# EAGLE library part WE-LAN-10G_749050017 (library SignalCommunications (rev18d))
WE-LAN 10G Transformer 10Gbit Base-T - Compliant with standards: IEEE 802.3an and upcoming IEEE 802.3bt - SMD -- Ethernet -- Ethernet speed up to 10Gbit/s --Power over Ethernet PoE and PoE+ --10Gbit with ETR and PoE up to 150 W (for industrial applications) Details see: http://katalog.we-online.de/en/pbs/WE-LAN-10G 2015 (C) Würth Elektronik
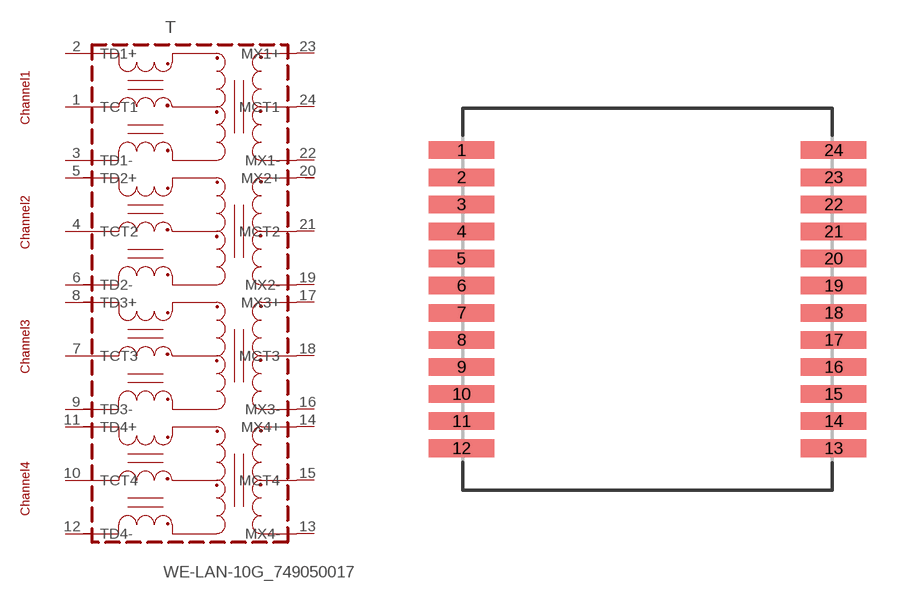
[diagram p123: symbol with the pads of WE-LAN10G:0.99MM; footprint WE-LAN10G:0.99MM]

Designator prefix T

## WE-LAN-10G_749050017  [WE-LAN10G:0.99MM]
1  TCT1
2  TD1+
3  TD1-
4  TCT2
5  TD2+
6  TD2-
7  TCT3
8  TD3+
9  TD3-
10  TCT4
11  TD4+
12  TD4-
13  MX4-
14  MX4+
15  MCT4
16  MX3-
17  MX3+
18  MCT3
19  MX2-
20  MX2+
21  MCT2
22  MX1-
23  MX1+
24  MCT1

## Footprint WE-LAN10G:0.99MM (pad centres in mm)
WE-LAN 10G:0.99mm
smd 2.4 x 0.64: 1 -6.8,5.445; 2 -6.8,4.455; 3 -6.8,3.465; 4 -6.8,2.475; 5 -6.8,1.485; 6 -6.8,0.495; 7 -6.8,-0.495; 8 -6.8,-1.485; 9 -6.8,-2.475; 10 -6.8,-3.465; 11 -6.8,-4.455; 12 -6.8,-5.445; 13 6.8,-5.445; 14 6.8,-4.455; 15 6.8,-3.465; 16 6.8,-2.475; 17 6.8,-1.485; 18 6.8,-0.495; 19 6.8,0.495; 20 6.8,1.485; 21 6.8,2.475; 22 6.8,3.465; 23 6.8,4.455; 24 6.8,5.445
